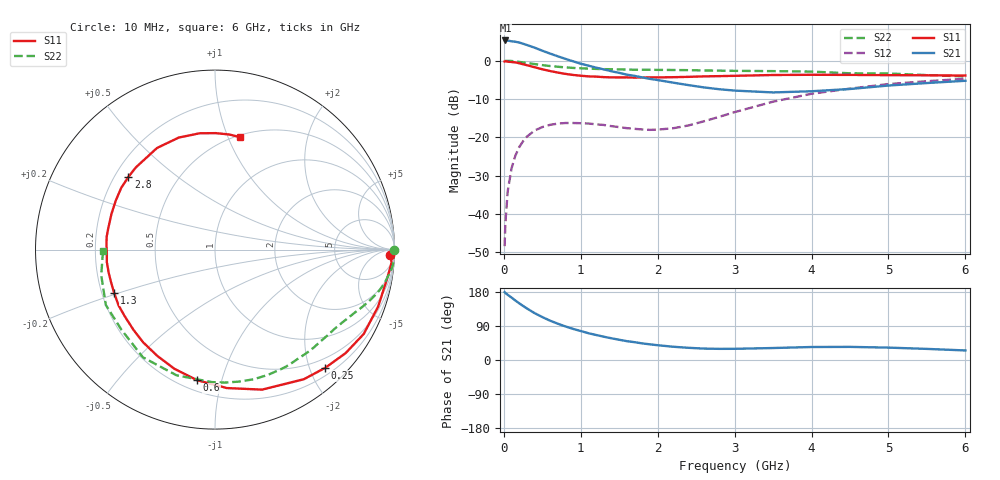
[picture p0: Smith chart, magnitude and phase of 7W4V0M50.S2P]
! Infineon Technologies  Discrete & RF Semiconductors
! BFS17W
! Si NPN RF Bipolar Junction Transistor in SOT323
! VCE = 4 V  IC = 0.5 mA
! Common Emitter S-Parameters:  August  1999
# GHz  S  MA  R  50
!  f  S11  S21  S12  S22
! GHz  MAG  ANG  MAG  ANG  MAG  ANG  MAG  ANG
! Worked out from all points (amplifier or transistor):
!   36 points, 10 MHz to 6 GHz, reference 50 ohm
!   highest |S21| = 5.3 dB at 20 MHz (marker M1)
!   |S21| within 3 dB of that: start of sweep to 543.7 MHz
!   unconditionally stable (mu >= 1): 1.225 GHz to end of sweep
!   at 250 MHz: K = 0.22, MSG = 12.7 dB, |S12| = -21.0 dB
!   at 1.4 GHz: K = 1.15, MAG = 4.8 dB, |S12| = -17.1 dB
!   at 6 GHz: K = 1.09, MAG = -2.1 dB, |S12| = -4.7 dB
!   S11 on the Smith chart (normalised r, x): 10 MHz: 30, -42; 250 MHz: 0.32, -2.26; 600 MHz: 0.26, -0.84; 1.3 GHz: 0.25, -0.19; 2.8 GHz: 0.26, +0.34; 6 GHz: 0.52, +1.11
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0.01  0.9776 -1.8  1.828 179.2  0.0038 90.1  0.9999 -0.1
0.02  0.9866 -4.2  1.841 177.0  0.0076 88.4  0.9966 -1.1
0.05  0.972 -9.8  1.832 172.1  0.0197 85.2  0.9962 -2.8
0.1  0.9627 -19.3  1.797 164.8  0.0394 78.3  0.9935 -5.5
0.15  0.9526 -29.6  1.771 156.9  0.0579 72.2  0.9796 -8.1
0.25  0.9006 -47.0  1.669 142.7  0.0891 61.9  0.9517 -12.8
0.3  0.8755 -55.6  1.606 136.0  0.1024 57.5  0.9372 -14.8
0.4  0.8232 -71.4  1.482 123.7  0.1229 49.1  0.9055 -18.5
0.5  0.7742 -85.1  1.353 113.3  0.1362 42.5  0.8775 -21.6
0.6  0.7345 -97.8  1.242 103.9  0.1457 37.2  0.8539 -24.3
0.8  0.6736 -118.6  1.059 88.6  0.154 29.3  0.8196 -29.4
1.1  0.6254 -143.4  0.863 70.7  0.1516 23.5  0.79 -36.7
1.3  0.6114 -156.9  0.771 61.4  0.1451 22.4  0.7775 -42.0
1.6  0.6066 -173.5  0.658 49.7  0.1319 25.3  0.7674 -49.9
2.2  0.6102 161.0  0.518 35.0  0.1315 46.4  0.7578 -67.2
2.8  0.6301 140.0  0.425 29.4  0.1854 63.2  0.7429 -85.7
3.5  0.6518 119.7  0.386 31.6  0.2925 64.3  0.7324 -107.0
4  0.6561 107.9  0.4 34.3  0.3707 58.6  0.722 -123.8
4.5  0.6537 97.5  0.428 34.6  0.4333 51.5  0.6863 -139.4
5  0.6489 89.6  0.475 32.7  0.4963 44.6  0.682 -153.1
5.5  0.6462 82.9  0.512 29.3  0.5412 37.6  0.6499 -167.2
6  0.6416 77.4  0.548 25.2  0.5818 31.2  0.6242 -179.4
